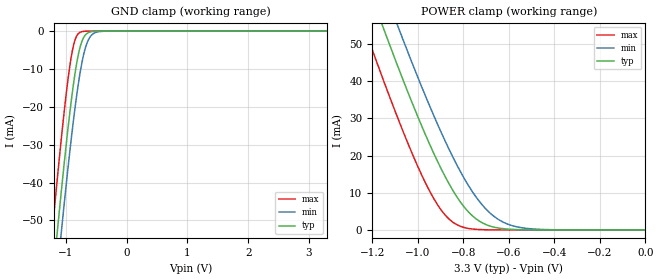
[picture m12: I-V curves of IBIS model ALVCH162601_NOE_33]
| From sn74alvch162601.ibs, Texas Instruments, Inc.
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[Model]   ALVCH162601_NOE_33
Model_type  Input
Vinl=0.8
Vinh=2.0
| variable   typ   min   max
C_comp   2.11pF   1.75pF   2.40pF
[Temperature Range]   40   100   -40
| Ambient temperature   25   85   -40
[Voltage range]   3.3   3   3.6
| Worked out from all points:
|   GND clamp passes 1 mA (typ) near -0.68 V on its own axis
|   POWER clamp passes 1 mA (typ) near -0.68 V on its own axis
[GND Clamp]
| ALVCH162601_NOE_33
|   Voltage   I(typ)   I(min)   I(max)
-3.3V     -451.4mA   -460.2mA   -440.6mA
-1.225V   -66.77mA   -77.63mA   -52.81mA
-1.14V    -52.55mA   -63.42mA   -38.55mA
-1.07V    -41.27mA   -52.08mA   -27.39mA
-975mV    -26.91mA   -37.4mA    -13.81mA
-905mV    -17.45mA   -27.36mA   -6.068mA
-845mV    -10.58mA   -19.54mA   -2.069mA
-765mV    -4.1mA     -10.78mA   -298.6uA
-700mV    -1.444mA   -5.604mA   -52.39uA
-640mV    -472.1uA   -2.617mA   -10.24uA
-470mV    -15.62uA   -178.3uA   -98.79nA
3.3V      1.114nA    9.952uA    5.63pA
[POWER Clamp]
| ALVCH162601_NOE_33
|   Voltage   I(typ)   I(min)   I(max)
-3.3V     451.4mA    460.2mA    440.6mA
-1.23V    67.62mA    78.48mA    53.67mA
-1.14V    52.55mA    63.42mA    38.55mA
-1.08V    42.85mA    53.67mA    28.94mA
-970mV    26.19mA    36.66mA    13.17mA
-880mV    14.42mA    24mA       4.064mA
-835mV    9.584mA    18.33mA    1.666mA
-775mV    4.712mA    11.75mA    387.5uA
-665mV    761.4uA    3.659mA    20.23uA
-595mV    194.7uA    1.357mA    2.999uA
-495mV    25.94uA    271uA      195.5nA
-48.03fV  1.114nA    59.61nA    6.941pA
